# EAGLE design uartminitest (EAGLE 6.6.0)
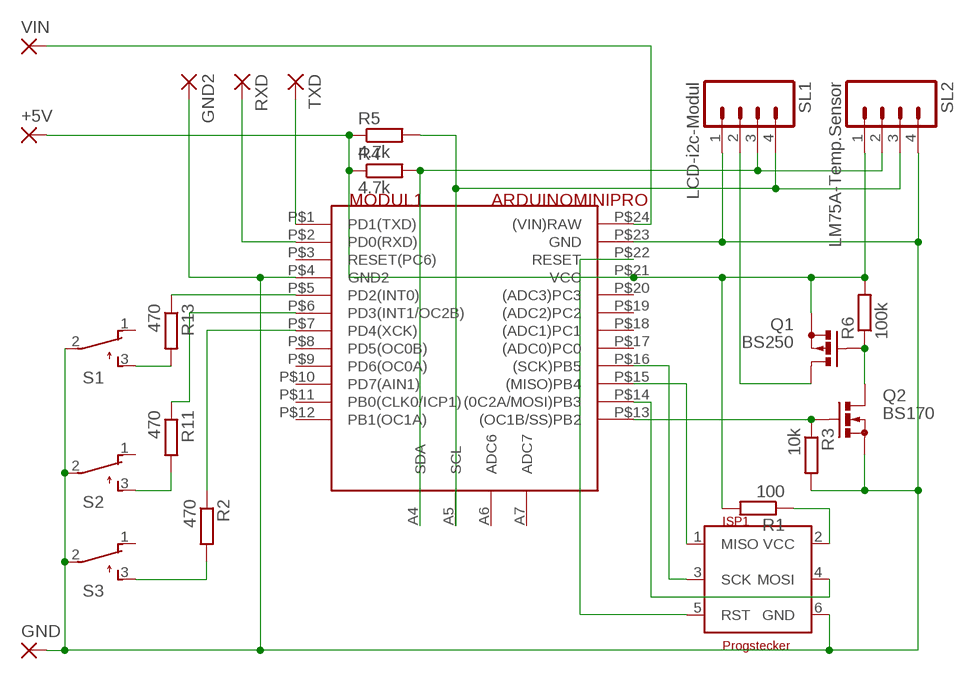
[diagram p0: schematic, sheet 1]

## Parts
+5V  2,54/1,0  [2,54/1,0]
GND  2,54/1,0  [2,54/1,0]
GND2  1,6/0,8  [1,6/0,8]
ISP1  Progstecker  ISP6N  [ISP6]
MODUL1  ARDUINOMINIPRO  [ARDUINOMINIPRO]
Q1  BS250  [SOT54E]
Q2  BS170  [SOT54E]
R1  100  R-EU_0204/5  [0204/5]
R2  470  R-EU_0204/7  [0204/7]
R3  10k  R-EU_0204/5  [0204/5]
R4  4.7k  R-EU_0204/7  [0204/7]
R5  4.7k  R-EU_0204/7  [0204/7]
R6  100k  R-EU_0204/5  [0204/5]
R11  470  R-EU_0204/7  [0204/7]
R13  470  R-EU_0204/7  [0204/7]
RXD  1,6/0,8  [1,6/0,8]
S1  TL32PO  [TL3XPO]
S2  TL32PO  [TL3XPO]
S3  TL32PO  [TL3XPO]
SL1  LCD-i2c-Modul  M04  [04P]
SL2  LM75A-Temp.Sensor  M04  [04P]
TXD  1,6/0,8  [1,6/0,8]
VIN  2,54/1,0  [2,54/1,0]

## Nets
GND [dick]: GND2.1(P) GND.1(P) ISP1.6(GND) MODUL1.P$4(GND2) MODUL1.P$23(GND) Q2.S R3.2 S1.2(P) S2.2(P) S3.2(P) SL1.1 SL2.4
N$1: ISP1.5(RST) MODUL1.P$22(RESET)
N$3: ISP1.3(SCK) MODUL1.P$16((SCK)PB5)
N$4: ISP1.1(MISO) MODUL1.P$15((MISO)PB4)
N$5: MODUL1.A4(SDA) R4.2 SL1.3 SL2.2
N$6: ISP1.4(MOSI) MODUL1.P$14((0C2A/MOSI)PB3)
N$7: MODUL1.P$1(PD1(TXD)) TXD.1(P)
N$8: MODUL1.P$2(PD0(RXD)) RXD.1(P)
N$9 [dick]: ISP1.2(VCC) R1.1
N$10: MODUL1.A5(SCL) R5.2 SL1.4 SL2.3
N$11: MODUL1.P$5(PD2(INT0)) R13.1
N$12: MODUL1.P$6(PD3(INT1/OC2B)) R11.1
N$13: R2.2 S3.3(S)
N$14: MODUL1.P$7(PD4(XCK)) R2.1
N$15: MODUL1.P$13((OC1B/SS)PB2) Q2.G R3.1
N$16 [dick]: Q1.G Q2.D R6.1
N$17 [dick]: Q1.D SL1.2
N$27: R11.2 S2.3(S)
N$53: R13.2 S1.3(S)
VCC [dick]: +5V.1(P) MODUL1.P$21(VCC) Q1.S R1.2 R4.1 R5.1 R6.2 SL2.1
VIN [dick2]: MODUL1.P$24((VIN)RAW) VIN.1(P)
Unconnected: MODUL1.A6(ADC6) MODUL1.A7(ADC7) MODUL1.P$3(RESET(PC6)) MODUL1.P$8(PD5(OC0B)) MODUL1.P$9(PD6(OC0A)) MODUL1.P$10(PD7(AIN1)) MODUL1.P$11(PB0(CLK0/ICP1)) MODUL1.P$12(PB1(OC1A)) MODUL1.P$17((ADC0)PC0) MODUL1.P$18((ADC1)PC1) MODUL1.P$19((ADC2)PC2) MODUL1.P$20((ADC3)PC3) S1.1(O) S2.1(O) S3.1(O)

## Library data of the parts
+5V GND VIN = wirepad:2,54/1,0: THROUGH-HOLE PAD
GND2 RXD TXD = wirepad:1,6/0,8: THROUGH-HOLE PAD
ISP1 = 6_stecker:ISP6: ISP-Stecker 6polig
MODUL1 = arduino:ARDUINOMINIPRO
Q1 = transistor-small-signal:BS250: P-CHANNEL MOS FET
Q2 = transistor-small-signal:BS170: N-CHANNEL MOS FET
R1-R6 R11 R13 = rcl:R-EU_: RESISTOR, European symbol
S1-S3 = switch:TL32PO: TINY SWITCH ON - MOM Source: http://www2.produktinfo.conrad.com/datenblaetter/700000-724999/705152-da-01-de-Subminiaturschalter_TL_36YO.pdf
SL1 SL2 = con-amp-quick:M04: AMP QUICK CONNECTOR; OC_FARNELL: unknown; OC_NEWARK: unknown

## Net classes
1 dick: width 0.508 mm
2 dick2: width 0.762 mm

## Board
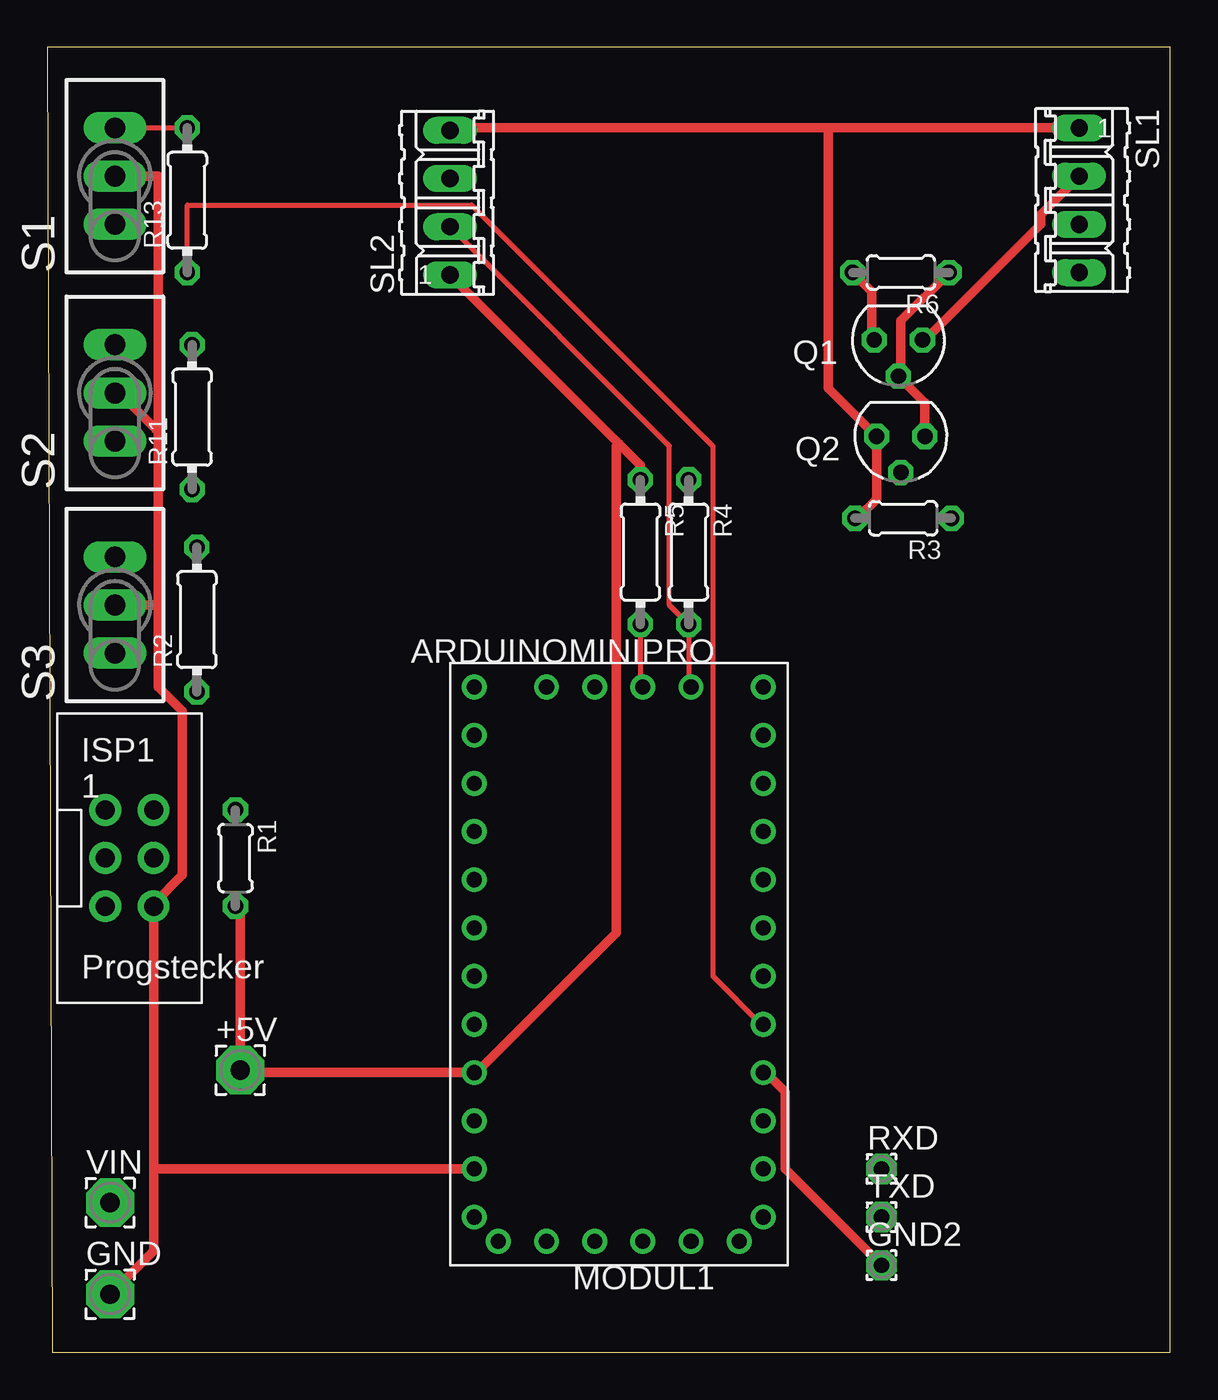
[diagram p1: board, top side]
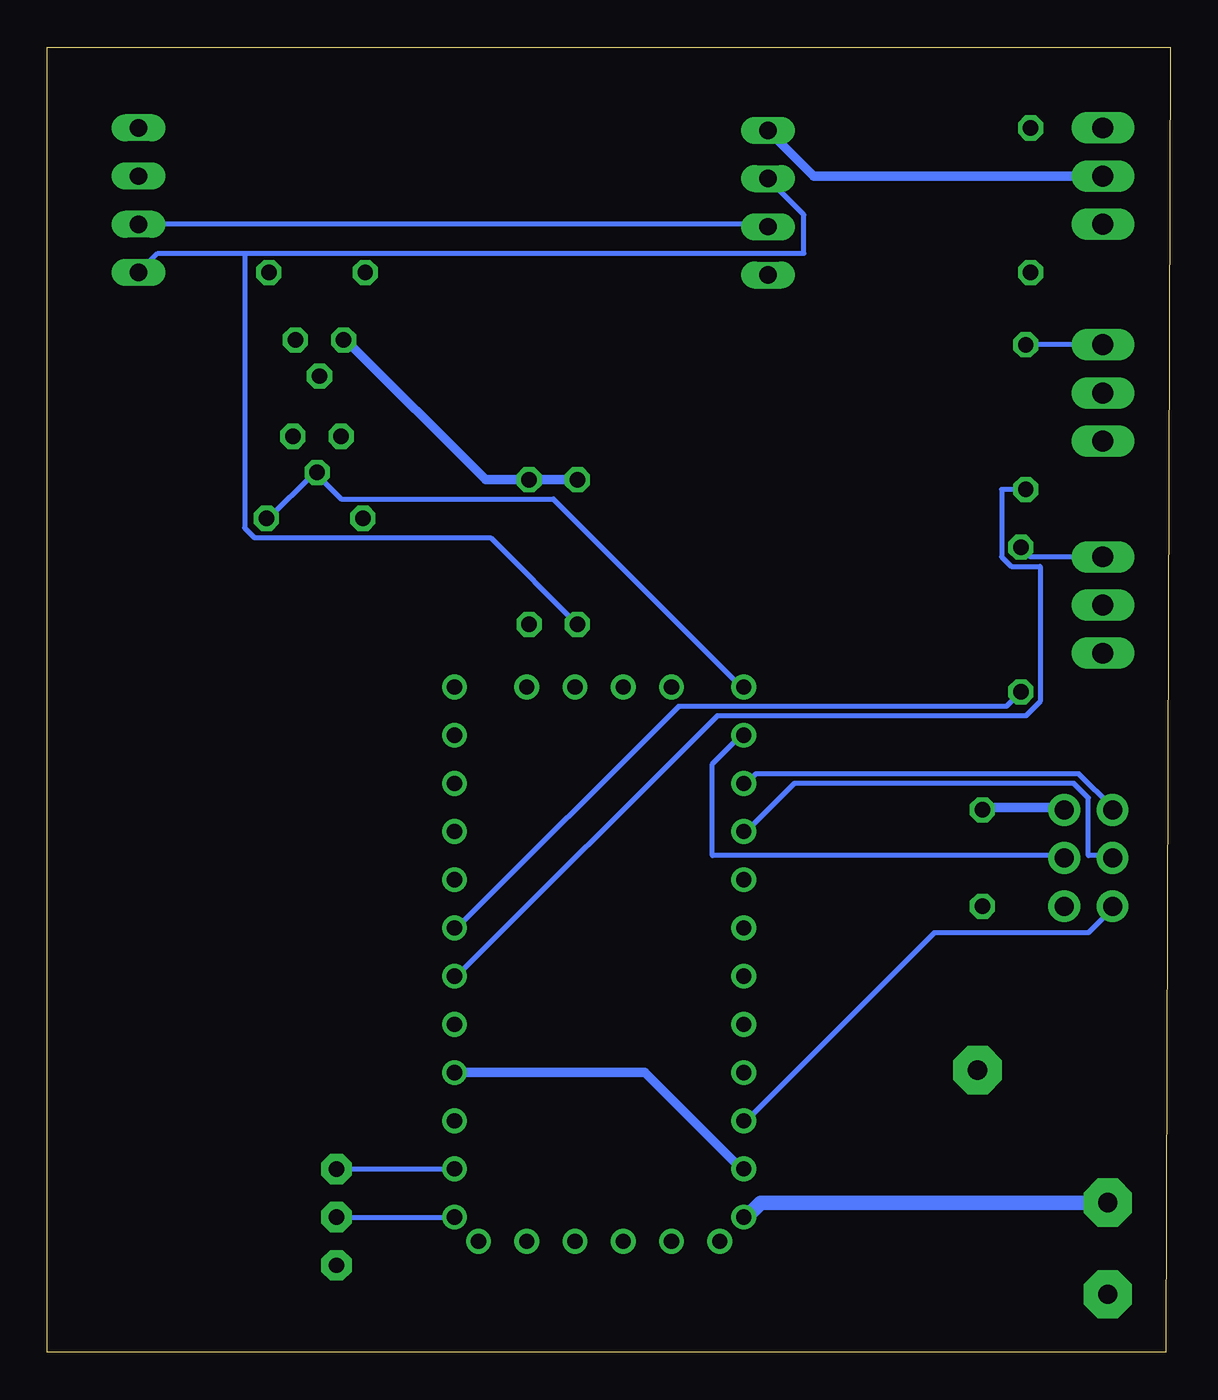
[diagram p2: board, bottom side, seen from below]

Size 59.16 x 68.76 mm. Coordinates in mm from the lower left corner, seen from the top.
Outline: 0.25,0 59.16,0 59.16,68.76 0,68.76 0.25,0
Copper layers (1*16): Top 0.035mm / dielectric 1.5mm / Bottom 0.035mm
Design rules "default": minimum track width 10mil, minimum drill 24mil, track to track 8mil, track to pad 8mil, pad to pad 8mil, via to via 8mil, smd to smd 8mil, copper to edge 40mil, drill to drill 8mil, minimum pad ring 10mil, minimum via ring 8mil, stop-mask expansion 4mil, vias tented up to drill 0mil, thermal gap 10mil

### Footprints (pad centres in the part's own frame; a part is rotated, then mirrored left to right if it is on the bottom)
2,54/1,0 = drill 1.016 pad 2.54 octagon: 1 0,0
1,6/0,8 = drill 0.813 pad 1.6 octagon: 1 0,0
ISP6 = drill 1 pad 1.676: 1 -1.27,2.54; 2 1.27,2.54; 3 -1.27,0; 4 1.27,0; 5 -1.27,-2.54; 6 1.27,-2.54
ARDUINOMINIPRO = drill 0.8: A4 -3.81,-13.97; A5 -1.27,-13.97; A6 1.27,-13.97; A7 3.81,-13.97; P$1 -7.62,13.97; P$2 -7.62,11.43; P$3 -7.62,8.89; P$4 -7.62,6.35; P$5 -7.62,3.81; P$6 -7.62,1.27; P$7 -7.62,-1.27; P$8 -7.62,-3.81; P$9 -7.62,-6.35; P$10 -7.62,-8.89; P$11 -7.62,-11.43; P$12 -7.62,-13.97; P$13 7.62,-13.97; P$14 7.62,-11.43; P$15 7.62,-8.89; P$16 7.62,-6.35; P$17 7.62,-3.81; P$18 7.62,-1.27; P$19 7.62,1.27; P$20 7.62,3.81; P$21 7.62,6.35; P$22 7.62,8.89; P$23 7.62,11.43; P$24 7.62,13.97; P$25 6.35,15.24; P$26 3.81,15.24; P$27 1.27,15.24; P$28 -1.27,15.24; P$29 -3.81,15.24; P$30 -6.35,15.24
SOT54E = drill 0.813 octagon: D -1.27,0; G 0,1.905; S 1.27,0
0204/5 = drill 0.813 octagon: 1 -2.54,0; 2 2.54,0
0204/7 = drill 0.813 octagon: 1 -3.81,0; 2 3.81,0
TL3XPO = drill 1.1 pad 1.422 long: 1 -2.54,0; 2 0,0; 3 2.54,0
04P = drill 0.914 long: 1 -3.81,0; 2 -1.27,0; 3 1.27,0; 4 3.81,0

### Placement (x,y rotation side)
+5V  10.16,14.86 0 top
GND  3.3,3.05 0 top
GND2  43.94,4.57 0 top
ISP1  4.32,26.04 0 top
MODUL1  30.1,21.08 180 top
Q1  44.83,53.34 180 top
Q2  44.96,48.26 180 top
R1  9.91,26.04 270 top
R2  7.87,38.61 90 top
R3  45.09,43.94 180 top
R4  33.78,42.16 270 top
R5  31.24,42.16 270 top
R6  44.96,56.9 180 top
R11  7.62,49.28 90 top
R13  7.37,60.71 90 top
RXD  43.94,9.65 0 top
S1  3.56,61.98 90 top
S2  3.56,50.55 90 top
S3  3.56,39.37 90 top
SL1  54.36,60.71 270 top
SL2  21.21,60.58 90 top
TXD  43.94,7.11 0 top
VIN  3.3,7.87 0 top

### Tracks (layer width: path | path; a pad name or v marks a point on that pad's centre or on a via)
GND
  Top 0.508: R3.2 42.67,43.94 43.69,44.96 Q2.S 41.15,50.8 41.15,64.52 | 41.15,64.52 21.34,64.52 SL2.4 | 41.15,64.52 SL1.1 | 22.61,9.65 MODUL1.P$23 5.59,9.65 | GND2.1 38.86,9.65 38.86,13.72 37.85,14.73 MODUL1.P$4 | 5.84,39.37 S3.2 | 5.84,39.37 5.84,48.51 5.71,48.64 | 5.71,48.64 3.81,50.55 S2.2 | 5.84,39.37 5.84,35.05 7.11,33.78 7.11,25.15 5.59,23.62 ISP1.6 5.59,9.65 | GND.1 5.59,5.33 5.59,9.65 | S1.2 5.84,61.98 5.84,48.77 5.71,48.64
  Bottom 0.508: SL2.4 18.8,61.98 S1.2 | MODUL1.P$4 27.69,14.73 22.61,9.65 MODUL1.P$23
N$1
  Bottom 0.254: MODUL1.P$22 22.35,12.19 12.45,22.1 4.32,22.1 3.05,23.37 ISP1.5
N$3
  Bottom 0.254: MODUL1.P$16 22.35,27.43 19.81,29.97 5.08,29.97 4.32,29.21 4.32,26.16 3.05,26.16 ISP1.3
N$4
  Bottom 0.254: MODUL1.P$15 22.35,29.97 21.84,30.48 4.83,30.48 3.05,28.7 ISP1.1
N$5
  Top 0.254: MODUL1.A4 33.78,35.05 R4.2 32.77,39.37 32.77,47.75 SL2.2
  Bottom 0.254: SL1.3 21.34,59.44 SL2.2
N$6
  Bottom 0.254: MODUL1.P$14 22.61,32.51 24.13,30.99 24.13,26.16 5.59,26.16 ISP1.4
N$7
  Bottom 0.254: TXD.1 MODUL1.P$1
N$8
  Bottom 0.254: RXD.1 MODUL1.P$2
N$9
  Bottom 0.508: R1.1 9.91,28.7 5.59,28.7 ISP1.2
N$10
  Top 0.254: R5.2 31.24,35.05 MODUL1.A5
  Bottom 0.254: SL2.3 19.3,59.94 19.3,57.91 48.77,57.91 | 48.77,57.91 53.34,57.91 SL1.4 | R5.2 35.81,42.93 48.26,42.93 48.77,43.43 48.77,57.91
N$11
  Top 0.254: R13.1 7.37,60.45 22.35,60.45 35.05,47.75 35.05,19.81 37.59,17.27 MODUL1.P$5
N$12
  Bottom 0.254: R11.1 8.89,45.47 8.89,41.91 8.38,41.4 6.86,41.4 6.86,34.29 7.62,33.53 23.88,33.53 37.59,19.81 MODUL1.P$6
N$13
  Bottom 0.254: R2.2 7.37,41.91 S3.3
N$14
  Bottom 0.254: R2.1 8.64,34.04 25.91,34.04 37.59,22.35 MODUL1.P$7
N$15
  Bottom 0.254: 44.96,46.23 43.69,44.96 32.51,44.96 22.61,35.05 MODUL1.P$13 | 44.96,46.23 45.21,46.23 47.5,43.94 R3.1 | 44.96,46.23 Q2.G
N$16
  Top 0.508: Q2.D 46.23,50.04 Q1.G 44.96,51.56 44.96,54.36 R6.1
N$17
  Top 0.508: SL1.2 52.32,59.94 52.32,59.44 46.23,53.34 Q1.D
N$27
  Bottom 0.254: S2.3 R11.2
N$53
  Top 0.254: S1.3 R13.2
VCC
  Top 0.508: R1.2 9.91,23.37 10.16,23.11 +5V.1 10.16,14.73 MODUL1.P$21 22.61,14.73 29.97,22.1 29.97,47.75 30.1,47.88 | R6.2 43.43,55.88 43.43,53.34 Q1.S | 30.1,47.88 31.24,46.74 R5.1 | 30.1,47.88 SL2.1
  Bottom 0.508: R5.1 R4.1 36.07,45.97 43.43,53.34 Q1.S
VIN
  Bottom 0.762: VIN.1 21.59,7.87 22.35,7.11 MODUL1.P$24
